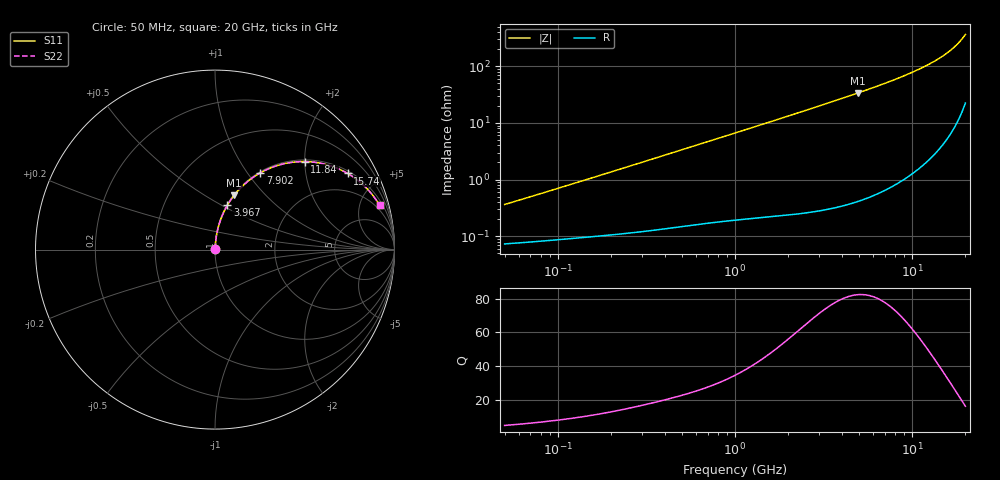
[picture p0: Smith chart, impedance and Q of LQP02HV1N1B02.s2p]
!Murata Part Number: LQP02HV1N1B02
!These Parameters are Measured in Series Mode Connection
!  o--[Z]--o
!Port1  Port2
!  o-------o
!Freq. Start=50[MHz] Stop=20[GHz], 401[Steps]
# Hz S RI R 50
!Freq.(Hz) S11(Real) S11(Imag) S21(Real) S21(Imag) S12(Real) S12(Imag) S22(Real) S22(Imag)
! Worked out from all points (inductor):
!   401 points, 50 MHz to 20 GHz, reference 50 ohm
!   read as one part in series: L = 1.12 nH near 51.52 MHz
!   highest Q = 82.4 at 4.967 GHz (marker M1), where L = 1.09 nH
!   S11 on the Smith chart (normalised r, x): 50 MHz: 1.00, +0.01; 3.967 GHz: 1.01, +0.53; 7.902 GHz: 1.02, +1.15; 11.84 GHz: 1.04, +2.00; 15.74 GHz: 1.10, +3.42; 20 GHz: 1.45, +7.28
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5e7  0.000741 0.00354  0.9993 -0.00354  0.9993 -0.00354  0.000741 0.00354
1.364002e8  0.00103 0.00935  0.999 -0.00935  0.999 -0.00935  0.00103 0.00935
3.721004e8  0.00193 0.0249  0.9981 -0.0249  0.9981 -0.0249  0.00193 0.0249
6.380365e8  0.00342 0.0423  0.9966 -0.0423  0.9966 -0.0423  0.00342 0.0423
1e9  0.00625 0.0657  0.9937 -0.0657  0.9937 -0.0657  0.00625 0.0657
1.714689e9  0.0148 0.1114  0.9852 -0.1114  0.9852 -0.1114  0.0148 0.1114
2.728004e9  0.0342 0.1746  0.9658 -0.1746  0.9658 -0.1746  0.0342 0.1746
3.967106e9  0.0693 0.2477  0.9307 -0.2477  0.9307 -0.2477  0.0693 0.2477
4.966507e9  0.1061 0.302  0.8939 -0.302  0.8939 -0.302  0.1061 0.302
6.125241e9  0.1576 0.3582  0.8424 -0.3582  0.8424 -0.3582  0.1576 0.3582
7.442007e9  0.226 0.4117  0.774 -0.4117  0.774 -0.4117  0.226 0.4117
7.901521e9  0.252 0.4274  0.748 -0.4274  0.748 -0.4274  0.252 0.4274
9.745021e9  0.3644 0.4735  0.6356 -0.4735  0.6356 -0.4735  0.3644 0.4735
1.082228e10  0.4341 0.487  0.5659 -0.487  0.5659 -0.487  0.4341 0.487
1.183995e10  0.5007 0.4905  0.4993 -0.4905  0.4993 -0.4905  0.5007 0.4905
1.375312e10  0.6233 0.4729  0.3767 -0.4729  0.3767 -0.4729  0.6233 0.4729
1.573793e10  0.7391 0.4243  0.2609 -0.4243  0.2609 -0.4243  0.7391 0.4243
1.670968e10  0.7892 0.391  0.2108 -0.391  0.2108 -0.391  0.7892 0.391
1.774144e10  0.8365 0.3502  0.1635 -0.3502  0.1635 -0.3502  0.8365 0.3502
1.855685e10  0.8694 0.3147  0.1306 -0.3147  0.1306 -0.3147  0.8694 0.3147
1.940974e10  0.8992 0.2751  0.1008 -0.2751  0.1008 -0.2751  0.8992 0.2751
2e10  0.9171 0.2467  0.0829 -0.2467  0.0829 -0.2467  0.9171 0.2467
